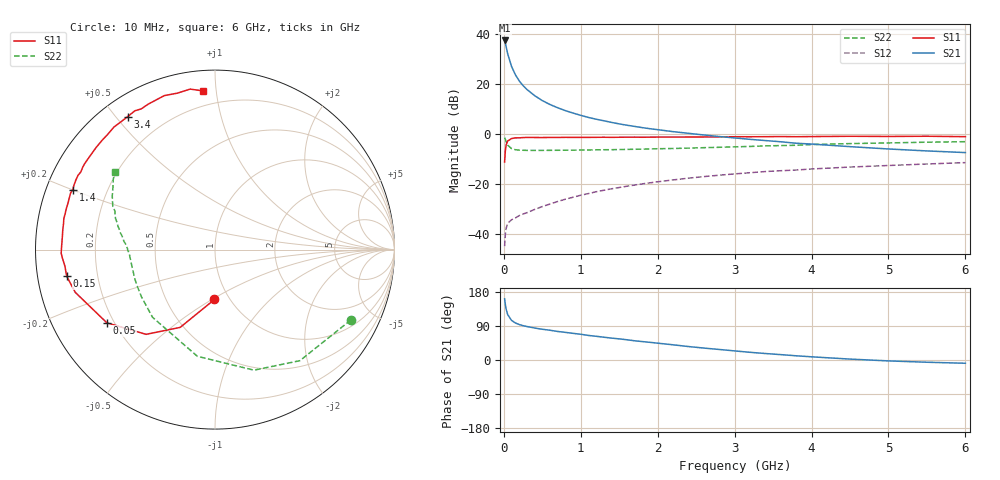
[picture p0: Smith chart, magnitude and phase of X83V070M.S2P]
! SIEMENS Small Signal Semiconductors
! BFP136W
! Si NPN RF Bipolar Junction Transistor in SOT343
! VCE = 3 V  IC = 70 mA
! Common Emitter S-Parameters:  September  1994
# GHz  S  MA  R  50
!  f  S11  S21  S12  S22
! GHz  MAG  ANG  MAG  ANG  MAG  ANG  MAG  ANG
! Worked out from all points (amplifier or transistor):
!   40 points, 10 MHz to 6 GHz, reference 50 ohm
!   highest |S21| = 37.4 dB at 10 MHz (marker M1)
!   |S21| within 3 dB of that: start of sweep to 33.39 MHz
!   unconditionally stable (mu >= 1): 557.2 MHz to 2.886 GHz
!   at 200 MHz: K = 0.62, MSG = 26.9 dB, |S12| = -32.5 dB
!   at 1.5 GHz: K = 1.10, MAG = 10.8 dB, |S12| = -21.3 dB
!   at 6 GHz: K = 0.97, MSG = 2.0 dB, |S12| = -11.4 dB
!   S11 on the Smith chart (normalised r, x): 10 MHz: 0.85, -0.51; 50 MHz: 0.17, -0.30; 150 MHz: 0.09, -0.09; 1.4 GHz: 0.08, +0.20; 3.4 GHz: 0.08, +0.54; 6 GHz: 0.11, +0.92
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0.01  0.2779 -90.6  73.73 161.5  0.0058 72.8  0.8525 -27.4
0.02  0.4746 -114.1  64.34 145.8  0.0102 59.3  0.7789 -52.6
0.03  0.6084 -129.1  55.11 134.2  0.0132 51.7  0.706 -72.1
0.05  0.7275 -145.9  40 119.8  0.0165 39.1  0.6024 -99.4
0.1  0.8143 -163.0  22.39 104.5  0.0195 34.2  0.5132 -132.7
0.15  0.8395 -169.8  15.27 97.7  0.0212 36.0  0.487 -147.2
0.2  0.8412 -173.7  11.48 93.6  0.0236 38.0  0.4787 -155.1
0.25  0.8514 -176.8  9.272 90.6  0.0254 40.9  0.4753 -160.2
0.3  0.8573 -178.7  7.756 88.4  0.027 43.8  0.4726 -163.6
0.4  0.854 177.5  5.843 84.4  0.0313 48.3  0.4722 -168.1
0.5  0.8535 174.8  4.654 81.1  0.0358 51.7  0.4727 -171.0
0.6  0.8551 172.7  3.886 78.5  0.0402 54.2  0.4736 -173.0
0.7  0.8565 170.1  3.349 75.3  0.0451 56.3  0.4751 -174.3
0.9  0.8583 166.6  2.622 70.3  0.0549 58.4  0.4776 -176.9
1.1  0.8591 162.2  2.145 64.8  0.065 59.5  0.4819 -178.5
1.4  0.8596 157.1  1.709 57.8  0.0809 59.6  0.488 179.2
2.2  0.8699 143.2  1.118 40.1  0.1217 55.0  0.5151 173.3
3.2  0.8841 126.3  0.785 20.3  0.1693 46.1  0.5666 164.5
3.4  0.8863 123.3  0.742 17.1  0.1789 44.0  0.5808 162.6
4.5  0.9032 108.2  0.561 2.4  0.2197 33.8  0.6454 152.5
5.5  0.9049 98.8  0.461 -5.9  0.253 26.0  0.6887 145.4
6  0.8874 94.5  0.427 -8.6  0.2693 21.6  0.705 142.3
